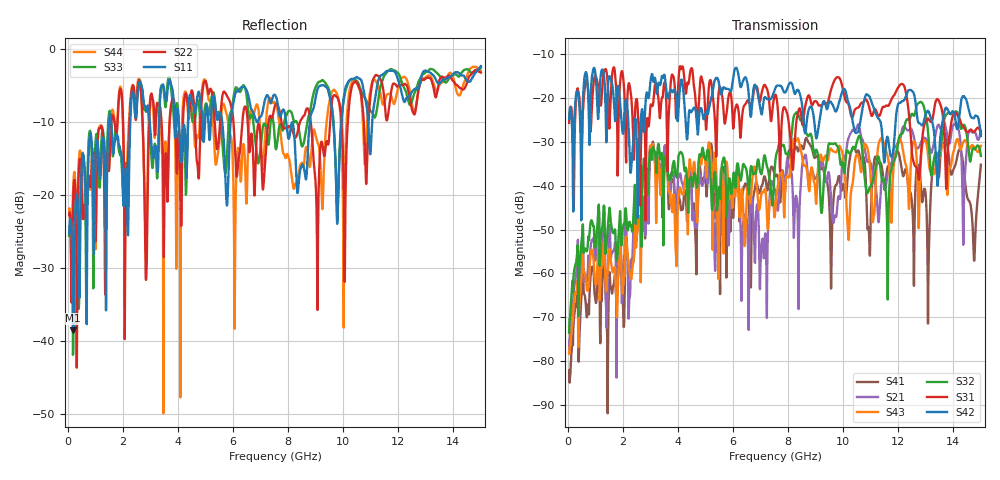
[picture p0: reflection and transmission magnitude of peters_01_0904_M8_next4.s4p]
# MHZ S RI R 50.00
! FREQ  S11  S12  S13  S14
!  S21  S22  S23  S24
!  S31  S32  S33  S34
!  S41  S42  S43  S44
!  REAL  IMAG  REAL  IMAG  REAL  IMAG  REAL  IMAG
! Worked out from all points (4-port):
!   1496 points, 50 MHz to 15 GHz, reference 50 ohm
!   strongest paths, dB at 50 MHz, 3.79 GHz, 7.53 GHz, 11.27 GHz, 15 GHz:
!     S42: -24.7, -18.6, -17.8, -24.6, -28.7
!     S31: -25.7, -14.6, -19.2, -24.0, -28.1
!     S32: -73.6, -36.7, -34.9, -33.3, -33.2
!     S43: -78.1, -45.9, -46.0, -31.1, -30.9
!     S21: -75.4, -37.6, -41.2, -47.6, -27.4
!     S41: -83.3, -39.1, -37.8, -34.9, -35.2
!   lowest |S11| = -38.6 dB at 200 MHz (marker M1), VSWR 1.02, Z = 48.9 + j0.326 ohm
!   |S11| at or under -10 dB: start of sweep to 1.5 GHz; 1.576 GHz to 2.27 GHz (694.1 MHz wide, 36.1 % of centre); 8.152 GHz to 8.787 GHz (635.2 MHz wide, 7.5 % of centre)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
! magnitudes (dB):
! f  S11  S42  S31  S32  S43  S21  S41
! 50 MHz  -25.3  -24.7  -25.7  -73.6  -78.1  -75.4  -83.3
! 200 MHz  -38.6  -45.9  -31.7  -61.5  -68.6  -66.4  -72.5
! 2.26 GHz  -11.2  -35.0  -17.5  -48.6  -60.5  -65.2  -59.2
! 3.06 GHz  -13.9  -14.5  -21.8  -33.6  -31.7  -32.4  -31.7
! 7.18 GHz  -6.7  -19.8  -17.2  -33.8  -41.1  -51.0  -38.4
! 8 GHz  -12.0  -17.4  -24.5  -33.0  -37.9  -34.7  -32.8
! 15 GHz  -2.3  -28.7  -28.1  -33.2  -30.9  -27.4  -35.2
